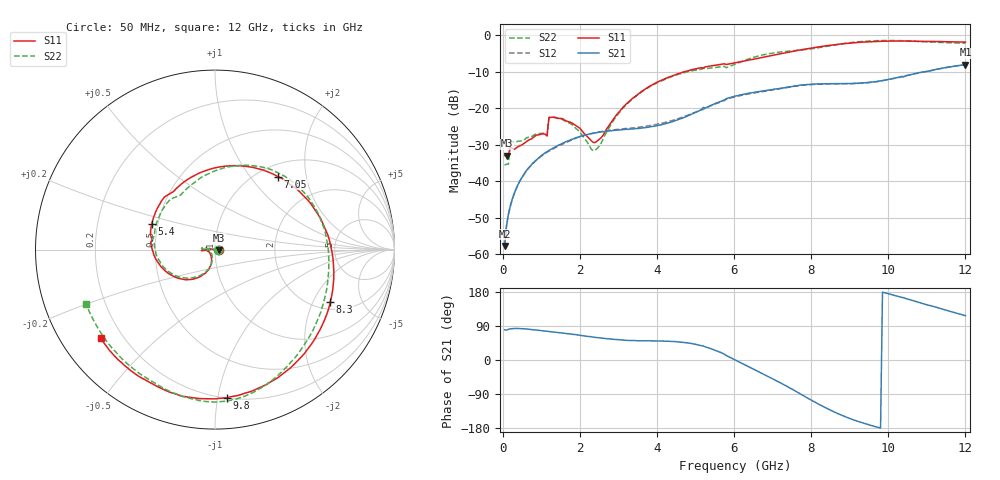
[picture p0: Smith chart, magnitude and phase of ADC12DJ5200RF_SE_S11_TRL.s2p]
#  HZ  S  DB  R  50.00
! Rohde & Schwarz ZVA24 4Ports - Version 3.90 - 1145.1110k26 SN: 100644
! Date: 2019-01-22 14:37:27
! Measurements: S11 S31 S13 S33
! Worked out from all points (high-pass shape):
!   240 points, 50 MHz to 12 GHz, reference 50 ohm
!   highest |S21| = -8.03 dB at 12 GHz (marker M1); lowest = -57.7 dB at 50 MHz (marker M2)
!   |S21| within 3 dB of the highest: 10.48 GHz to end of sweep
!   lowest |S11| = -33.0 dB at 100 MHz (marker M3), VSWR 1.05, Z = 52.3 - j0.335 ohm
!   |S11| at or under -10 dB: start of sweep to 4.71 GHz
!   |S22| runs from -35.6 to -1.4 dB; largest |S21 - S12| = 0.013
!   S11 on the Smith chart (normalised r, x): 50 MHz: 1.05, -0.00; 5.4 GHz: 0.46, +0.15; 7.05 GHz: 1.21, +1.39; 8.3 GHz: 2.34, -2.74; 9.8 GHz: 0.20, -1.06; 12 GHz: 0.12, -0.34
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5e7  -32.96 -5.1  -57.70 79.6  -57.78 78.4  -35.57 -4.2
1e8  -32.96 -8.2  -52.25 78.8  -52.09 81.6  -35.32 -9.4
1.5e8  -32.76 -12.2  -48.87 80.9  -49.15 81.9  -35.32 -14.8
2e8  -30.66 169.9  -46.65 82.3  -46.83 82.6  -29.29 167.7
6.5e8  -28.89 -172.0  -36.59 81.6  -36.69 81.5  -27.98 -177.9
1.15e9  -27.55 -177.6  -31.87 75.8  -32.05 75.9  -27.59 -174.9
1.2e9  -22.55 -175.1  -31.55 75.1  -31.77 75.4  -22.50 175.4
2.05e9  -26.07 -176.4  -27.58 64.6  -27.61 66.8  -27.21 171.0
2.4e9  -29.36 -146.5  -26.75 59.7  -26.70 61.7  -31.43 -147.1
3.1e9  -19.96 -106.5  -25.87 52.7  -25.68 54.2  -20.19 -105.4
4.05e9  -12.65 -133.9  -24.67 50.1  -24.28 49.7  -12.78 -136.4
5.4e9  -8.40 158.0  -19.24 29.9  -19.30 27.8  -8.95 157.1
6.05e9  -7.52 110.7  -16.61 -0.8  -16.80 -1.8  -7.79 101.4
6.55e9  -6.47 79.7  -15.57 -26.3  -15.75 -26.6  -5.91 67.8
7.05e9  -5.40 49.2  -14.75 -52.2  -14.87 -52.4  -4.81 40.5
8.05e9  -3.43 -10.7  -13.40 -108.5  -13.47 -108.4  -3.64 -18.1
8.3e9  -3.02 -24.6  -13.32 -122.2  -13.38 -122.1  -3.22 -33.3
8.95e9  -2.19 -55.5  -13.21 -152.4  -13.27 -152.2  -2.11 -63.8
9.8e9  -1.64 -85.4  -12.49 -179.5  -12.53 -179.4  -1.44 -85.6
1.005e10  -1.59 -93.0  -12.01 173.6  -12.04 173.8  -1.43 -91.4
1.105e10  -1.68 -119.8  -9.81 144.6  -9.83 144.8  -1.84 -120.6
1.2e10  -1.88 -142.2  -8.03 117.0  -8.04 117.2  -2.15 -157.1
